(* Logix 5000 AddOnInstructionDefinition export MAHSP_Yaskawa; software revision 17.00 *)

TYPE Yaskawa_EIP_Servo :   // Yaskawa SigmaLogic Axis Structure v2.4.0
STRUCT
   O : Yaskawa_OUT_to_Servo;
   I : Yaskawa_IN_from_Servo;
   AOI_SB : Yaskawa_AOI_Status_Bits;
END_STRUCT
END_TYPE

TYPE Yaskawa_OUT_to_Servo :   // Structure of data sent out to the Yaskawa SigmaLogic controller v2.4.0
STRUCT
   b00_ServoOn : BOOL;   // Servo On
   b01_Stop : BOOL;   // Stops All Current Motion in Progress
   b02_Home : BOOL;   // Start Homing Process
   b03_MoveStart1 : BOOL;   // Start Current Motion
   b06_SuperImpose : BOOL;
   b07_ServoAlarmReset : BOOL;   // Servo Alarm Reset
   b08_ControllerAlarmReset : BOOL;   // SigmaLogic Alarm Reset
   b09_MoveStart2 : BOOL;   // Start Second Motion (Blended Move)
   b10_MoveAbort : BOOL;   // Abort Current Move
   b11_MovePause : BOOL;   // Pause Current Move
   b12_SeqPause : BOOL;   // Indexing Sequence Pause
   b13_SeqResume : BOOL;   // Indexing Sequence Resume
   b14_SeqCancel : BOOL;   // Indexing Sequence Cancel
   b15_AbsEncoderReset : BOOL;   // Absolute Encoder Reset
   b16_SeqStart : BOOL;   // Start Indexing Sequence
   b17_SeqEditSpeed : BOOL;   // Enter Edit Speed
   b18_SeqEditDistance : BOOL;   // Enter Distance Edit
   b19_PLSEnable : BOOL;   // Enable PLS execution
   b20_PLSActivateOutput1 : BOOL;   // Activate PLS output1 switch logic
   b21_PLSActivateOutput2 : BOOL;   // Activate PLS output2 switch logic
   b22_PLSActivateOutput3 : BOOL;   // Activate PLS output3 switch logic
   b23_PLSActivateOutput4 : BOOL;   // Activate PLS output4 switch logic
   b24_SetClock : BOOL;   // Set the remote controller clock with data provided by the PLC
   RebootController : BOOL;
   UseExternalEncoder : BOOL;   // Use External Encoder when executing MAHSP_Yaskawa
   b32_HeatbeatAnswer : BOOL;   // Heartbeat Answer
   BrakeBypassRequest : BOOL;
   SetFwdTorqueLimit : BOOL;
   SetRevTorqueLimit : BOOL;
   TorqueLimit : DINT;
   TorqueRamp : DINT;
   HomeMethod : INT;
   HomeSpeed : DINT;
   HomeAccDec : DINT;   // Home Move Acceleration/Deceleration Rate
   HomeBackOffDistance : DINT;
   HomeCreepSpeed : DINT;
   HomeCreepDistanceLimit : DINT;
   HomeCreepTimeLimit : DINT;
   HomeOffsetDistance : DINT;
   HomeOffsetSpeed : DINT;
   HomePostion : DINT;
   HomeTorque : DINT;
   HomeInputNo : DINT;
   HomeApproachTimeLimit : DINT;
   HomeApproachDistLimit : DINT;
   HomeDirection : INT;
   HomeSwitchMode : INT;
   MoveType : INT;
   MoveDirection : INT;
   MoveAccel1 : DINT;
   MoveAccel2 : DINT;
   MoveDecel1 : DINT;
   MoveDecel2 : DINT;
   MoveSpeed1 : DINT;
   MoveSpeed2 : DINT;
   MoveDistance1 : DINT;
   MoveDistance2 : DINT;
   MovePosition1 : DINT;
   MovePosition2 : DINT;
   RegistrationDistance : DINT;
   GearNumerator : DINT;
   GearDenominator : DINT;
   SuperImposeDistance : DINT;
   Resolution : INT;
   RegistrationDirection : INT;
   TuningLevel : INT;
   SequenceStep : INT;   // Staring Sequence Step Number
   SequenceEditStep : INT;   // Sequence Step Number to Edit
   FlagCommandBits1 : DINT;   // Flag Commands. 1..64 are General Flags, Bits 0..31 correspond to Flag 1..32
   FlagCommandBits2 : DINT;   // Flag Commands cont. 1..64 are General Flags, Bits 0..31 correspond to Flag 33..64
   DigitalOutCommandBits : DINT;   // Digital Output commands. Bits 0-7 correspond to CN13 Digital Outputs 0-7, used as Flag 73-80. Bits 8-10 correspond to CN1 Digital Outputs 0-2 used as Flag 88-90"
   SequenceEditSpeed : DINT;
   SequenceEditDistance : DINT;
   FeedRateOverride : INT;
   HSI_Enable : BOOL;
   HSI_MoveMode : BOOL;   // 0=Relative; 1=Moves per Cycle
   HSI_CalcMethod : BOOL;   // 0=Accel/Decel; 1=Time
   HSI_MoveDirection : BOOL;   // 0 = Negative; 1 = Positive
   HSI_TriggerFlag : INT;
   HSI_MovingFlag : INT;
   HSI_DwellingFlag : INT;
   HSI_DoneFlag : INT;
   HSI_MoveType : INT;   // 0=Single; 1=Repeat; 2=Repeat "x" times
   HSI_RepeatNumber : INT;
   HSI_Distance : DINT;
   HSI_Speed : DINT;
   HSI_Accel : DINT;
   HSI_MoveTime : DINT;
   HSI_DwellTime : DINT;
   PLS_OutputFlag1 : INT;
   PLS_OutputFlag2 : INT;
   PLS_OutputFlag3 : INT;
   PLS_OutputFlag4 : INT;
   PLS_OnPosition1 : DINT;
   PLS_OffPosition1 : DINT;
   PLS_OnPosition2 : DINT;
   PLS_OffPosition2 : DINT;
   PLS_OnPosition3 : DINT;
   PLS_OffPosition3 : DINT;
   PLS_OnPosition4 : DINT;
   PLS_OffPosition4 : DINT;
   PLS_OnCompensation1 : INT;
   PLS_OffCompensation1 : INT;
   PLS_OnCompensation2 : INT;
   PLS_OffCompensation2 : INT;
   PLS_OnCompensation3 : INT;
   PLS_OffCompensation3 : INT;
   PLS_OnCompensation4 : INT;
   PLS_OffCompensation4 : INT;
   RTC_Year : INT;
   RTC_Month : INT;
   RTC_Day : INT;
   RTC_Hour : INT;
   RTC_Min : INT;
   RTC_Sec : INT;
   StopDecel : DINT;
   AnalogOutput : INT;   // CN13, AO_01 [mV]
END_STRUCT
END_TYPE

TYPE Yaskawa_AOI_Status_Bits :   // Internal bits used to interlock Yaskawa AOI execution. v2.4.0
STRUCT
   MAM : BOOL;   // Move AOI Active
   MAJ : BOOL;   // Jog AOI Active
   MAB : BOOL;   // Blending AOI Active
   MAG : BOOL;   // Gearing AOI Active
   MAHSP : BOOL;   // Home SetPoint AOI Active
   MAH : BOOL;   // Homing AOI Active
   MSQE : BOOL;   // Sequence Edit AOI Active
   MSQR : BOOL;   // Sequence Run AOI Active
   MHSI : BOOL;   // High Speed Index AOI Active
   MSO : BOOL;   // Servo On
   MSF : BOOL;   // Servo Off
   MAFR : BOOL;   // Fault Reset
   MAS : BOOL;   // Servo Abort
   MTRQ : BOOL;   // Torque Mode Active
   MPLS : BOOL;   // PLS Active
   MCLK : BOOL;   // SetClock Active
   MSTL : BOOL;   // Set Torque Limit Active
   AOI_Permissive : BOOL;   // Permissive to Execute an AOI
END_STRUCT
END_TYPE

TYPE Yaskawa_IN_from_Servo :   // Structure of data coming from the Yaskawa SigmaLogic controller. v2.4.0
STRUCT
   AlarmText : STRING;   // ServoPack Alarm Code plus Text Description
   b00_Heartbeat : BOOL;
   b01_Alarm : BOOL;   // ServoPack Alarm
   b02_Warning : BOOL;   // ServoPack Warning
   b03_Ready : BOOL;   // ServoPack Ready
   b04_Enabled : BOOL;   // ServoPack Enabled ("Servo On")
   b05_StopComplete : BOOL;
   b06_HomeComplete : BOOL;
   b07_HomeBusy : BOOL;
   b08_HomeActive : BOOL;
   b09_HomeAborted : BOOL;
   b10_HomeError : BOOL;
   b11_MoveAbsComplete : BOOL;
   b12_MoveAbsBusy : BOOL;
   b13_MoveAbsActive : BOOL;
   b14_MoveAbsAborted : BOOL;
   b15_MoveAbsError : BOOL;
   b16_MoveRelComplete : BOOL;
   b17_MoveRelBusy : BOOL;
   b18_MoveRelActive : BOOL;
   b19_MoveRelAborted : BOOL;
   b20_MoveRelError : BOOL;
   b21_JogAtSpeed : BOOL;
   b22_JogBusy : BOOL;
   b23_JogActive : BOOL;
   b24_JogAborted : BOOL;
   b25_JogError : BOOL;
   b26_GearInSync : BOOL;
   b27_GearBusy : BOOL;
   b28_GearActive : BOOL;
   b29_GearAborted : BOOL;
   b30_GearError : BOOL;
   b32_MoveSuperComplete : BOOL;
   b33_MoveSuperBusy : BOOL;
   b34_MoveSuperActive : BOOL;
   b35_MoveSuperAborted : BOOL;
   b36_MoveSuperError : BOOL;
   b37_PowerCycleRequired : BOOL;
   b38_MoveBlend1Complete : BOOL;
   b39_MoveBlend1Busy : BOOL;
   b40_MoveBlend1Active : BOOL;
   b41_MoveBlend1Abort : BOOL;
   b42_MoveBlend1Error : BOOL;
   b43_MoveBlend2Complete : BOOL;
   b44_MoveBlend2Busy : BOOL;
   b45_MoveBlend2Active : BOOL;
   b46_MoveBlend2Abort : BOOL;
   b47_MoveBlend2Error : BOOL;
   b48_RegComplete : BOOL;
   b49_RegBusy : BOOL;
   b50_RegActive : BOOL;
   b51_RegAborted : BOOL;
   b52_RegError : BOOL;
   b53_ResetAbsEncoderActive : BOOL;
   b54_ResetAbsEncoderBusy : BOOL;
   b55_ResetAbsEncoderDone : BOOL;
   b56_ResetAbsEncoderError : BOOL;
   b57_SeqRunning : BOOL;
   b58_RegSensorNotReached : BOOL;
   b59_SeqEditError : BOOL;
   b60_SeqEditDone : BOOL;
   b61_TorqueAtTorque : BOOL;
   b62_TorqueBusy : BOOL;
   b63_TorqueActive : BOOL;
   b64_TorqueAborted : BOOL;
   b65_TorqueError : BOOL;
   b66_ControllerAlarm : BOOL;
   b67_ApplicationError : BOOL;
   b68_AxisAtStandStill : BOOL;
   b69_TestModeActive : BOOL;
   b70_ServoParamsOK : BOOL;
   b71_SetFwdTorqueLimitDone : BOOL;
   b72_SetRevTorqueLimitDone : BOOL;
   Position : DINT;
   Speed : DINT;
   Torque : DINT;
   HomeErrorID : INT;
   MoveAbsErrorID : INT;
   MoveRelErrorID : INT;
   JogErrorID : INT;
   GearErrorID : INT;
   MoveSuperErrorID : INT;
   ServoAlarmID : INT;
   ServoWarningID : INT;
   ControllerAlarmID : DINT;
   AxisGenAlarmID : DINT;
   MoveBlend1ErrorID : INT;
   MoveBlend2ErrorID : INT;
   ResetAbsEncoderErrorID : INT;
   FunctionBlockErrorID : INT;
   TorqueErrorID : INT;
   RegErrorID : INT;
   SeqCurrentStep : INT;
   FlagStatusBit1 : DINT;   // Flag Status. 1..64 are General Flags, Bits 0..31 correspond to Flag 1..32
   FlagStatusBit2 : DINT;   // Flag Status cont. 1..64 are General Flags, Bits 0..31 correspond to Flag 33..64
   IOStatusBits : DINT;   // Digital IO Status. Bits 0-7, CN13 Inputs 0-7, Used as Flag 65-72. Bits 8-15, CN13 Outputs 0-7, Used as Flag 73-80. Bits 16-22, CN1 Inputs 0-6, Used as Flag 81-87. Bits 23-25, CN1 Outputs 0-4, Used as Flag 88-92.
   HSI_Moving : BOOL;
   HSI_Dwelling : BOOL;
   HSI_Done : BOOL;
   HSI_Busy : BOOL;
   HSI_Error : BOOL;
   HSI_ErrorCode : INT;
   PLS_Running : BOOL;
   PLS_SwitchStatus1 : BOOL;
   PLS_SwitchStatus2 : BOOL;
   PLS_SwitchStatus3 : BOOL;
   PLS_SwitchStatus4 : BOOL;
   PLS_Busy : BOOL;
   PLS_Error : BOOL;
   PLS_ErrorCode : INT;
   SetClock_Done : BOOL;
   SetClock_Busy : BOOL;
   SetClock_Error : BOOL;
   SetClock_ErrorID : INT;
   SoftwareVersion : DINT;
   FirmwareVersion : DINT;
   CommandedPos : DINT;
   CommandedPosNonCyc : DINT;
   CommandedSpeed : DINT;
   Clock_Year : INT;
   Clock_Month : INT;
   Clock_Day : INT;
   Clock_Hour : INT;
   Clock_Minute : INT;
   Clock_Second : INT;
   AnalogInput : REAL;   // CN13, AI_01 [v]
   BrakeBypassActive : BOOL;
   ForwardTorqueLimit : DINT;
   ReverseTorqueLimit : DINT;
END_STRUCT
END_TYPE

ADD_ON_INSTRUCTION MAHSP_Yaskawa   (* revision 2.4 0, vendor Yaskawa America, Inc., ExecuteEnableInFalse *)
// Motion Axis Home "Set Position"
// Revision note:
// 2.4.0: No functional change.
// 2.3.1: Moved unlatch of AOI_ON_LOCAL to bottom of EnableInFalse routine so that outputs will be on for at least 1 scan if one-shot on EN is used.
// 2.3.0: No functional change
// 2.0.0: Improved output operation and error code reporting. Improved interlocking with embedded code. Added input for UseExternalEncoder
// 1.2.0: No functional change.
// Initial Release 9/10/2014
// Help:
// This AOI sets the current position of the servo motor or of the External Encoder (if applicable) to a specified value. This command is a simpler alternative to the MAH_Yaskawa command with HomeType = 0. Axis can be in either an enabled or disabled state.
VAR_IN_OUT
   Axis : Yaskawa_EIP_Servo; {required}
END_VAR
VAR_INPUT
   SetPosition : REAL; {required}   // Set the current position to this value
   UseExternalEncoder : INT; {required}   // If set to 1, the Set Position will apply to the external encoder axis instead of the main motor axis
END_VAR
VAR_OUTPUT
   ErrorCode : INT; {visible}   // Set Position Error Code
   EN : BOOL; {visible}   // The AOI is Active
   DN : BOOL; {visible}   // Homing is Completed
   ER : BOOL; {visible}   // Homing Process Error
   FLT_BSY : BOOL; {visible}   // There is another AOI Active for this Axis
   FLT_RDY : BOOL; {visible}   // The Servo is Not Ready
   IP : BOOL;   // Homing is In Process
END_VAR
VAR
   AOI_ON_LOCAL : BOOL;
   ScaleFactor : DINT;
   Finished : BOOL;   // Function is Finished
   Debug1 : BOOL;
END_VAR

ROUTINE EnableInFalse   (* ladder *)
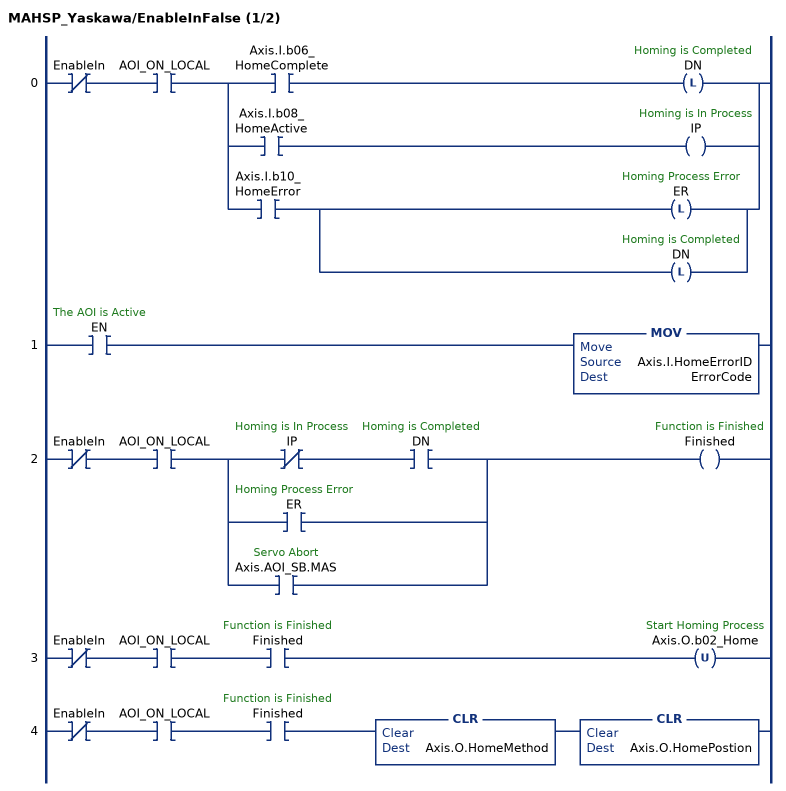
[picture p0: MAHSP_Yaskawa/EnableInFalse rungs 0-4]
   0: XIO(EnableIn)XIC(AOI_ON_LOCAL)[XIC(Axis.I.b06_HomeComplete) OTL(DN) ,XIC(Axis.I.b08_HomeActive) OTE(IP) ,XIC(Axis.I.b10_HomeError) [OTL(ER) ,OTL(DN) ] ];
   1: XIC(EN)MOV(Axis.I.HomeErrorID,ErrorCode);
   2: XIO(EnableIn)XIC(AOI_ON_LOCAL)[XIO(IP) XIC(DN) ,XIC(ER) ,XIC(Axis.AOI_SB.MAS) ]OTE(Finished);
   3: XIO(EnableIn)XIC(AOI_ON_LOCAL)XIC(Finished)OTU(Axis.O.b02_Home);
   4: XIO(EnableIn)XIC(AOI_ON_LOCAL)XIC(Finished)CLR(Axis.O.HomeMethod)CLR(Axis.O.HomePostion);
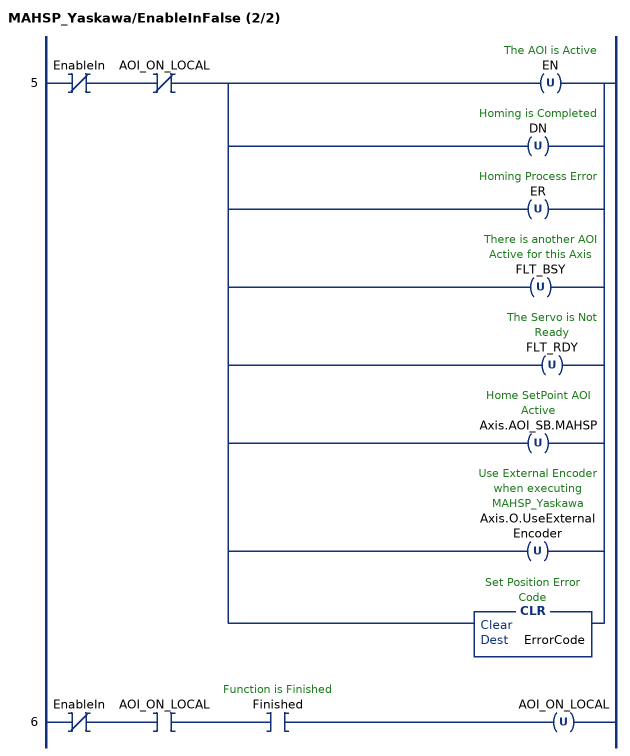
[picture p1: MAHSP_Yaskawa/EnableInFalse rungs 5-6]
   5: XIO(EnableIn)XIO(AOI_ON_LOCAL)[OTU(EN) ,OTU(DN) ,OTU(ER) ,OTU(FLT_BSY) ,OTU(FLT_RDY) ,OTU(Axis.AOI_SB.MAHSP) ,OTU(Axis.O.UseExternalEncoder) ,CLR(ErrorCode) ];
   6: XIO(EnableIn)XIC(AOI_ON_LOCAL)XIC(Finished)OTU(AOI_ON_LOCAL);
END_ROUTINE

ROUTINE Logic   (* ladder *)
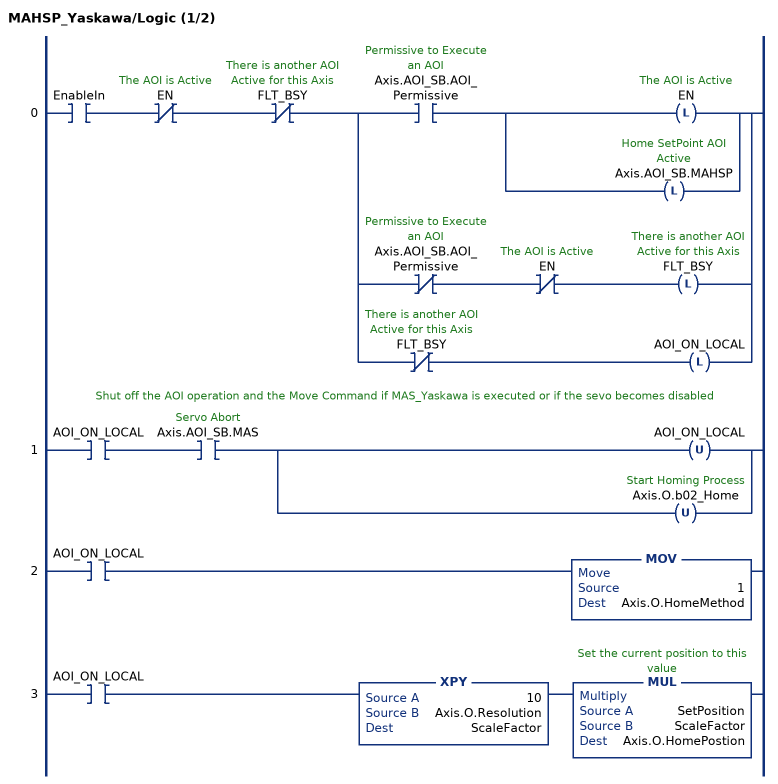
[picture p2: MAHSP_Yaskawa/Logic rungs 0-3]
   0: XIC(EnableIn)XIO(EN)XIO(FLT_BSY)[XIC(Axis.AOI_SB.AOI_Permissive) [OTL(EN) ,OTL(Axis.AOI_SB.MAHSP) ] ,XIO(Axis.AOI_SB.AOI_Permissive) XIO(EN) OTL(FLT_BSY) ,XIO(FLT_BSY) OTL(AOI_ON_LOCAL) ];
   // Shut off the AOI operation and the Move Command if MAS_Yaskawa is executed or if the sevo becomes disabled
   1: XIC(AOI_ON_LOCAL)XIC(Axis.AOI_SB.MAS)[OTU(AOI_ON_LOCAL) ,OTU(Axis.O.b02_Home) ];
   2: XIC(AOI_ON_LOCAL)MOV(1,Axis.O.HomeMethod);
   3: XIC(AOI_ON_LOCAL)XPY(10,Axis.O.Resolution,ScaleFactor)MUL(SetPosition,ScaleFactor,Axis.O.HomePostion);
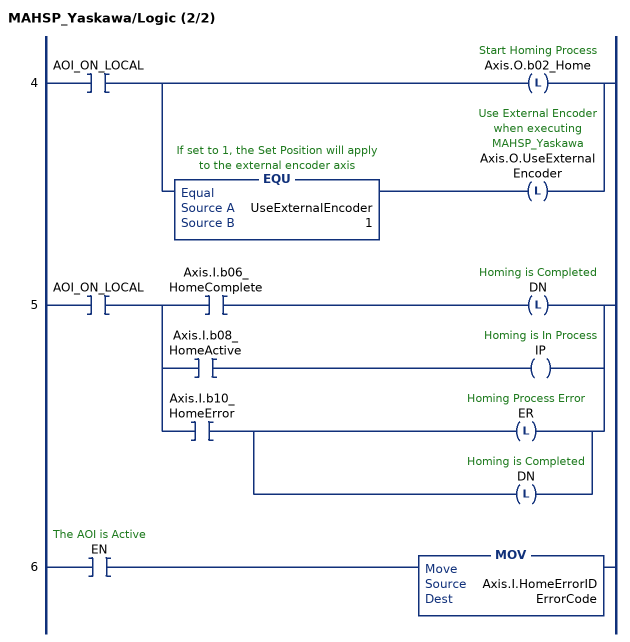
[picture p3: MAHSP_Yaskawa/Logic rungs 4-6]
   4: XIC(AOI_ON_LOCAL)[OTL(Axis.O.b02_Home) ,EQU(UseExternalEncoder,1) OTL(Axis.O.UseExternalEncoder) ];
   5: XIC(AOI_ON_LOCAL)[XIC(Axis.I.b06_HomeComplete) OTL(DN) ,XIC(Axis.I.b08_HomeActive) OTE(IP) ,XIC(Axis.I.b10_HomeError) [OTL(ER) ,OTL(DN) ] ];
   6: XIC(EN)MOV(Axis.I.HomeErrorID,ErrorCode);
END_ROUTINE
END_ADD_ON_INSTRUCTION
